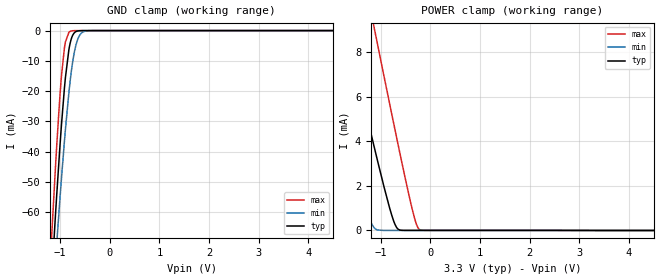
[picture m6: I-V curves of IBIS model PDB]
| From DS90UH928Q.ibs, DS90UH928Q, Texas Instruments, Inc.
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|   Model
[Model]   PDB
Model_type   Input
Vinl = 0.8
Vinh = 2.0
|   typ   min   max
C_comp   0.8892pF   0.8437pF   0.9472pF
[Voltage Range]   3.3   3   3.6
[Temperature Range]   25   105   -40
[Power Clamp Reference]   3.3   3   3.6
[GND Clamp Reference]   -0   -0   -0
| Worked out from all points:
|   GND clamp passes 1 mA (typ) near -0.73 V on its own axis
|   POWER clamp passes 1 mA (typ) near -0.82 V on its own axis
[GND Clamp]
|   Voltage   I(typ)   I(min)   I(max)
-3.3V     -715.7mA   -646.3mA   -779.6mA
-1.181V   -84.49mA   -97.09mA   -70.84mA
-1.092V   -60.18mA   -75.6mA    -44.2mA
-1.073V   -55mA      -70.95mA   -38.66mA
-1.013V   -40.13mA   -57.37mA   -23.39mA
-973.5mV  -30.97mA   -48.7mA    -14.82mA
-894.3mV  -15.45mA   -32.62mA   -3.717mA
-795.3mV  -3.886mA   -16.13mA   -228.9uA
-726mV    -948.4uA   -8.122mA   -22.91uA
-656.7mV  -172.3uA   -3.351mA   -6.055uA
-478.5mV  -3.688uA   -125.5uA   -3.699uA
6.59V     0A         0A         0A
[POWER Clamp]
|   Voltage   I(typ)   I(min)   I(max)
-3.3V     24.72mA    17.34mA    33.28mA
-2.518V   17.07mA    10.75mA    24.51mA
-2.251V   14.47mA    8.522mA    21.52mA
-1.716V   9.287mA    4.131mA    15.56mA
-1.27V    5.033mA    773.3uA    10.61mA
-1.122V   3.645mA    93.87uA    8.972mA
-1.082V   3.28mA     35.73uA    8.536mA
-825mV    1.028mA    2.141uA    5.72mA
-686.4mV  150.6uA    2.038uA    4.223mA
-359.7mV  3.746uA    1.866uA    889uA
-211.2mV  3.624uA    1.807uA    31.14uA
6.59V     0A         0A         0A
